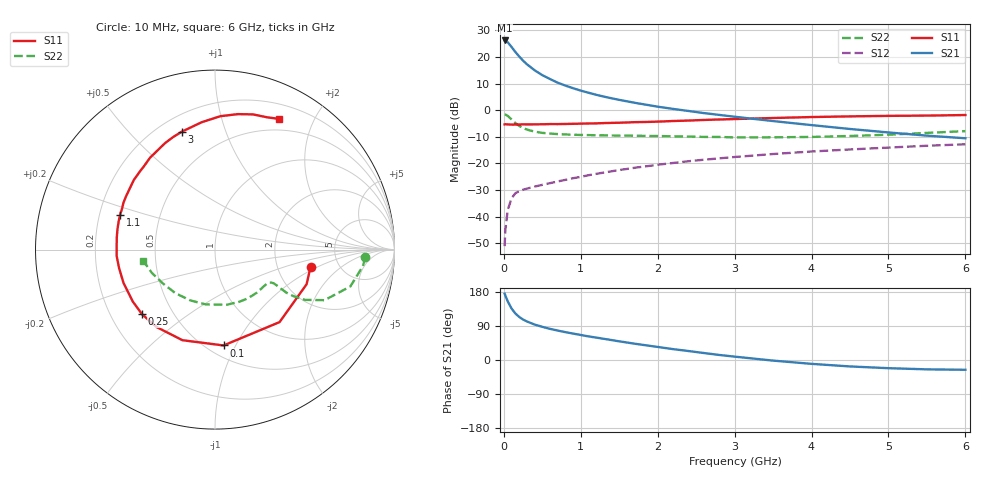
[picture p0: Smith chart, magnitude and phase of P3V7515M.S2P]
! SIEMENS Small Signal Semiconductors
! BFP181
! Si NPN RF Bipolar Junction Transistor in SOT143
! VCE = 0.75 V  IC = 15 mA
! Common Emitter S-Parameters:  March  1996
# GHz  S  MA  R  50
!  f  S11  S21  S12  S22
! GHz  MAG  ANG  MAG  ANG  MAG  ANG  MAG  ANG
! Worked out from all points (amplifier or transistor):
!   36 points, 10 MHz to 6 GHz, reference 50 ohm
!   highest |S21| = 26.2 dB at 10 MHz (marker M1)
!   |S21| within 3 dB of that: start of sweep to 114.9 MHz
!   unconditionally stable (mu >= 1): start of sweep to 19.37 MHz; 261.2 MHz to end of sweep
!   at 250 MHz: K = 0.97, MSG = 24.2 dB, |S12| = -29.9 dB
!   at 1.4 GHz: K = 2.34, MAG = 7.2 dB, |S12| = -22.9 dB
!   at 6 GHz: K = 2.17, MAG = -5.0 dB, |S12| = -12.8 dB
!   S11 on the Smith chart (normalised r, x): 10 MHz: 3.10, -0.85; 100 MHz: 0.60, -0.90; 250 MHz: 0.33, -0.34; 1.1 GHz: 0.29, +0.16; 3 GHz: 0.29, +0.71; 6 GHz: 0.36, +1.55
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0.01  0.5411 -10.3  20.39 174.9  0.0028 79.3  0.838 -3.0
0.02  0.5456 -20.7  20.26 169.9  0.0057 77.8  0.8295 -6.3
0.05  0.5409 -48.3  18.89 154.9  0.0133 70.4  0.7818 -15.2
0.1  0.5362 -84.9  15.4 136.0  0.0221 53.9  0.6721 -24.8
0.15  0.5364 -109.8  12.4 122.7  0.0276 46.9  0.5739 -29.2
0.2  0.5405 -127.1  10.19 113.6  0.0303 42.2  0.5077 -30.7
0.25  0.543 -138.4  8.508 106.8  0.0321 39.9  0.4639 -31.1
0.3  0.5418 -147.6  7.285 101.7  0.0337 39.6  0.4329 -30.7
0.4  0.5426 -160.1  5.621 93.5  0.0368 40.2  0.3955 -30.1
0.5  0.5443 -169.2  4.547 87.5  0.0397 40.4  0.3752 -29.9
0.6  0.5489 -176.1  3.849 82.2  0.0427 42.5  0.3642 -30.3
0.7  0.5483 177.6  3.285 77.7  0.0459 44.1  0.3561 -31.0
0.9  0.5552 168.2  2.587 69.8  0.0529 46.1  0.3465 -33.4
1.1  0.5633 159.9  2.13 62.3  0.0601 48.0  0.3407 -36.7
1.5  0.5817 146.0  1.563 49.2  0.0753 49.0  0.3346 -44.2
1.8  0.5992 136.5  1.304 40.1  0.0866 48.5  0.3301 -51.1
2.2  0.6267 125.3  1.057 28.7  0.1021 46.7  0.3228 -60.9
3  0.6823 105.8  0.754 8.9  0.1322 41.1  0.3087 -83.4
3.5  0.7134 96.0  0.625 -1.6  0.1504 37.2  0.3098 -99.6
4.5  0.7655 80.4  0.444 -17.0  0.1832 27.9  0.328 -132.3
5.5  0.792 68.6  0.333 -24.7  0.2151 19.0  0.3748 -159.7
6  0.8112 63.8  0.297 -25.8  0.2291 13.9  0.4048 -171.1
